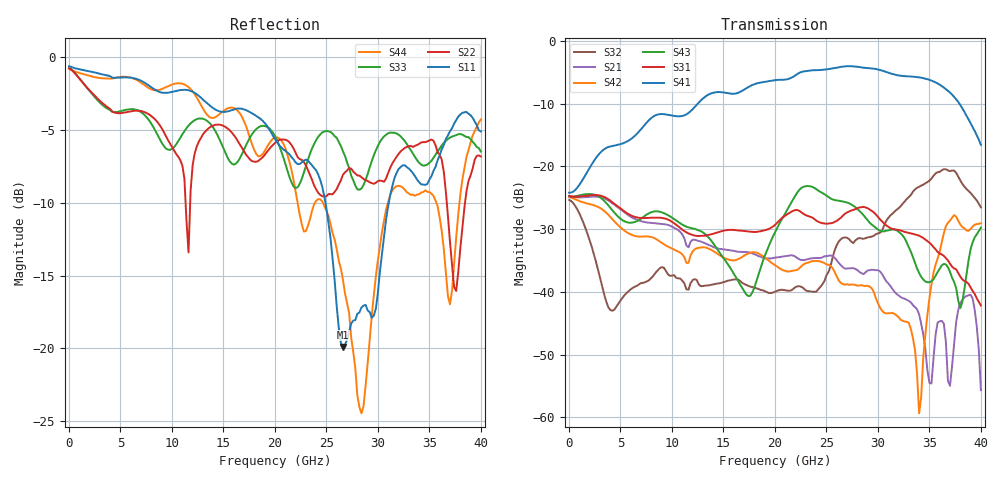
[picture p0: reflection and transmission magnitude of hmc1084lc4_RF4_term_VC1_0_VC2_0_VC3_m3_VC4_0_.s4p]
!Agilent Technologies,N5224A,MY51441122,A.09.40.06
!Agilent N5224A: A.09.40.06
!Date: Thursday, June 19, 2014 00:55:20
!Correction: S11(Full 4 Port(1,2,3,4))
!S12(Full 4 Port(1,2,3,4))
!S13(Full 4 Port(1,2,3,4))
!S14(Full 4 Port(1,2,3,4))
!S21(Full 4 Port(1,2,3,4))
!S22(Full 4 Port(1,2,3,4))
!S23(Full 4 Port(1,2,3,4))
!S24(Full 4 Port(1,2,3,4))
!S31(Full 4 Port(1,2,3,4))
!S32(Full 4 Port(1,2,3,4))
!S33(Full 4 Port(1,2,3,4))
!S34(Full 4 Port(1,2,3,4))
!S41(Full 4 Port(1,2,3,4))
!S42(Full 4 Port(1,2,3,4))
!S43(Full 4 Port(1,2,3,4))
!S44(Full 4 Port(1,2,3,4))
!S4P File: Measurements: <S11,S12,S13,S14>,
!<S21,S22,S23,S24>,
!<S31,S32,S33,S34>,
!<S41,S42,S43,S44>:
# Hz S  dB  R 50
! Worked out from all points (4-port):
!   201 points, 10 MHz to 40 GHz, reference 50 ohm
!   strongest paths, dB at 10 MHz, 10.01 GHz, 20 GHz, 30 GHz, 40 GHz:
!     S41: -24.2, -11.9, -6.3, -4.6, -16.6
!     S31: -24.7, -28.8, -29.3, -28.1, -42.2
!     S43: -24.8, -28.2, -30.5, -30.1, -29.8
!     S42: -24.9, -33.1, -35.8, -41.8, -29.1
!     S21: -24.8, -29.6, -34.6, -36.5, -55.6
!     S32: -25.4, -37.4, -40.0, -30.7, -26.5
!   lowest |S11| = -19.9 dB at 26.6 GHz (marker M1), VSWR 1.23, Z = 47.6 + j9.64 ohm
!   |S11| at or under -10 dB: 24.91 GHz to 31.06 GHz (6.15 GHz wide, 22 % of centre)
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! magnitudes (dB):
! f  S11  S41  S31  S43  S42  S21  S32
! 10 MHz  -0.6  -24.2  -24.7  -24.8  -24.9  -24.8  -25.4
! 4.209 GHz  -1.4  -16.8  -25.7  -27.0  -28.4  -25.9  -43.0
! 17.41 GHz  -3.7  -7.4  -30.4  -40.7  -33.9  -33.7  -39.0
! 26.6 GHz  -19.9  -4.1  -27.8  -25.6  -38.8  -36.1  -31.4
! 34 GHz  -8.6  -5.8  -31.0  -37.0  -59.3  -43.6  -23.2
! 36.6 GHz  -5.6  -7.7  -34.6  -35.6  -29.6  -48.0  -20.5
! 40 GHz  -5.1  -16.6  -42.2  -29.8  -29.1  -55.6  -26.5
